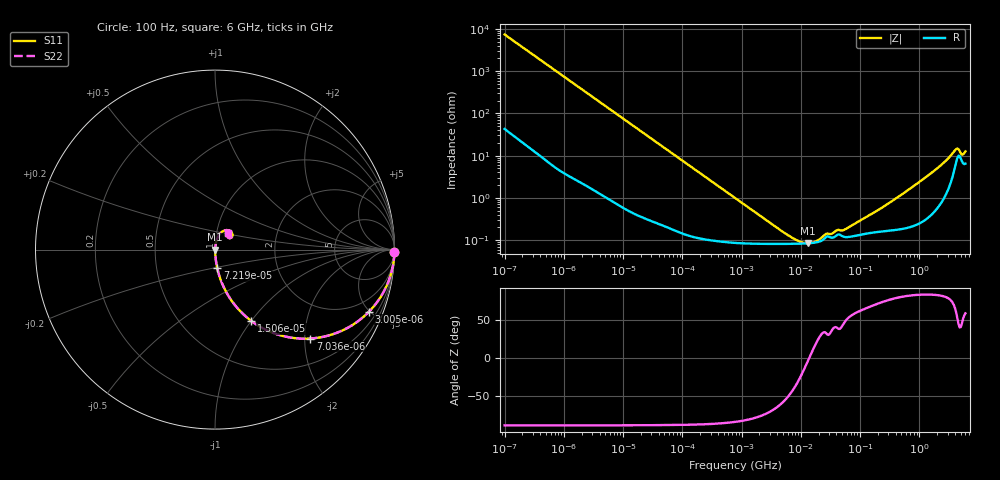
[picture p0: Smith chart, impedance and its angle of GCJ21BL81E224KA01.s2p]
!Murata Part Number: GCJ21BL81E224KA01
!These Parameters are Measured in Series Mode Connection
!Data Generated on Mar 13, 2026
!  o--ll--o
!Port1  Port2
!  o------o
!Operation Temp=25[degC], DC Bias Voltage=0[V]
!Freq. Start=100[Hz] Stop=6[GHz] 401[Steps]
# Hz S RI R 50
!Freq.(Hz) S11(Real) S11(Imag) S21(Real) S21(Imag) S12(Real) S12(Imag) S22(Real) S22(Imag)
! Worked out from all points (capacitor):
!   401 points, 100 Hz to 6 GHz, reference 50 ohm
!   read as one part in series: C = 215 nF near 109 Hz
!   lowest |Z| = 84.6 mohm at 13.01 MHz (marker M1)
!   series resonance near 13.87 MHz, so ESL is about 610 pH
!   S11 on the Smith chart (normalised r, x): 100 Hz: open; 3.005 kHz: 1.03, -4.96; 7.036 kHz: 1.02, -2.13; 15.06 kHz: 1.01, -1.00; 72.19 kHz: 1.00, -0.21; 6 GHz: 1.13, +0.22
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100  0.9997 -0.0136  0.000263 0.0136  0.000263 0.0136  0.9997 -0.0136
600  0.9931 -0.0802  0.00689 0.0802  0.00689 0.0802  0.9931 -0.0802
2008  0.9309 -0.2507  0.0691 0.2507  0.0691 0.2507  0.9309 -0.2507
3005  0.8587 -0.3451  0.1413 0.3451  0.1413 0.3451  0.8587 -0.3451
7036  0.5306 -0.4954  0.4694 0.4954  0.4694 0.4954  0.5306 -0.4954
15062  0.201 -0.3965  0.799 0.3965  0.799 0.3965  0.201 -0.3965
23569  0.0948 -0.2879  0.9052 0.2879  0.9052 0.2879  0.0948 -0.2879
40335  0.036 -0.1798  0.964 0.1798  0.964 0.1798  0.036 -0.1798
72189  0.0126 -0.1034  0.9874 0.1034  0.9874 0.1034  0.0126 -0.1034
774597  0.000958 -0.00985  0.999 0.00985  0.999 0.00985  0.000958 -0.00985
6353432  0.000818 -0.000958  0.9992 0.000958  0.9992 0.000958  0.000818 -0.000958
9506416  0.000826 -0.000432  0.9992 0.000432  0.9992 0.000432  0.000826 -0.000432
1.300572e7  0.000843 -7.23e-05  0.9992 7.23e-05  0.9992 7.23e-05  0.000843 -7.23e-05
1.555665e7  0.00086 0.000132  0.9991 -0.000132  0.9991 -0.000132  0.00086 0.000132
2.662322e7  0.00118 0.000769  0.9988 -0.000769  0.9988 -0.000769  0.00118 0.000769
5.699437e7  0.00119 0.00138  0.9988 -0.00138  0.9988 -0.00138  0.00119 0.00138
3.124326e8  0.00173 0.00741  0.9983 -0.00741  0.9983 -0.00741  0.00173 0.00741
1.712697e9  0.00607 0.0413  0.9939 -0.0413  0.9939 -0.0413  0.00607 0.0413
4.009986e9  0.064 0.1089  0.936 -0.1089  0.936 -0.1089  0.064 0.1089
4.385646e9  0.0919 0.0984  0.9081 -0.0984  0.9081 -0.0984  0.0919 0.0984
5.245841e9  0.0732 0.066  0.9268 -0.066  0.9268 -0.066  0.0732 0.066
6e9  0.0702 0.0947  0.9298 -0.0947  0.9298 -0.0947  0.0702 0.0947
